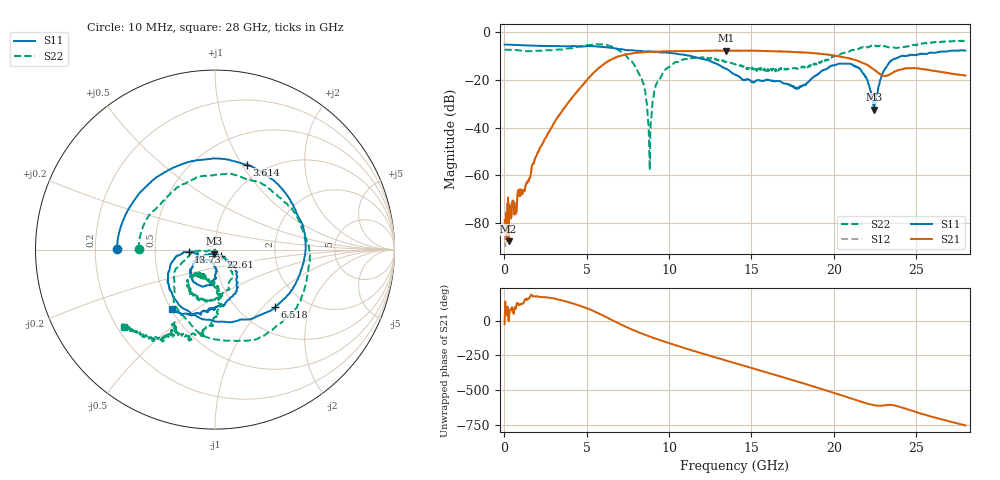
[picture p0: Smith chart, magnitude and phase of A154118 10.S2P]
!  2-Port S-parameters saved by WinCal
! VAR MeasName=S-Parameters (CALIBRATED_DATA) read from VNA (N5230A)
! VAR MeasDate=2015-9-10 14:35:09
! VAR NAME=A154118 10
! VAR FILENAME=A154118 10.S2P
! VAR DATE=2015-9-10 14:35:09
! VAR PHYS_PORTS=1,2
# Hz S DB R 50
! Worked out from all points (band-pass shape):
!   801 points, 10 MHz to 28 GHz, reference 50 ohm
!   highest |S21| = -7.79 dB at 13.45 GHz (marker M1); lowest = -87.6 dB at 254.9 MHz (marker M2)
!   |S21| within 3 dB of the highest: 6.716 GHz to 20.77 GHz (14.05 GHz wide, 102 % of centre)
!   lowest |S11| = -32.6 dB at 22.44 GHz (marker M3), VSWR 1.05, Z = 49.3 - j2.21 ohm
!   |S11| at or under -10 dB: 11.27 GHz to 24.14 GHz (12.87 GHz wide, 72.7 % of centre); 24.27452 GHz to 24.36083 GHz (86.3 MHz wide, 0.355 % of centre); 24.36195 GHz to 24.42704 GHz (65.09 MHz wide, 0.267 % of centre)
!   |S22| runs from -57.8 to -3.5 dB; largest |S21 - S12| = 0.0071
!   S11 on the Smith chart (normalised r, x): 10 MHz: 0.30, +0.00; 3.614 GHz: 0.83, +1.05; 6.518 GHz: 1.44, -1.17; 13.73 GHz: 0.74, -0.02; 22.61 GHz: 1.06, -0.08; 28 GHz: 0.51, -0.40
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1e7  -5.29 179.6  -78.78 -25.4  -79.54 -24.8  -7.49 179.8
2.549125e8  -5.29 172.2  -87.62 -2.1  -75.94 71.4  -7.44 172.1
3.613712e9  -5.94 69.5  -32.06 143.0  -32.03 143.0  -7.25 62.7
4.698325e9  -6.04 27.7  -22.61 103.5  -22.56 103.3  -6.00 12.5
5.573012e9  -6.03 -7.9  -16.06 60.8  -16.04 60.8  -5.06 -35.4
6.517675e9  -6.68 -43.8  -11.44 5.3  -11.43 5.1  -6.08 -91.9
8.302038e9  -7.94 -90.1  -8.59 -90.9  -8.52 -91.1  -19.42 -176.6
8.82685e9  -8.12 -100.8  -8.36 -114.7  -8.28 -114.9  -57.83 -47.6
9.10675e9  -8.32 -106.8  -8.26 -126.8  -8.21 -127.2  -24.36 -42.6
9.351662e9  -8.46 -111.7  -8.27 -136.9  -8.20 -137.2  -20.75 -39.0
1.089111e10  -9.52 -139.5  -8.02 163.5  -7.98 162.7  -11.50 -83.1
1.34452e10  -15.29 -175.3  -7.79 72.9  -7.77 72.4  -12.63 -130.1
1.37251e10  -16.60 -174.8  -7.82 63.1  -7.82 62.3  -12.86 -131.5
1.4005e10  -17.83 -175.1  -7.84 53.4  -7.81 53.0  -13.50 -132.7
1.603428e10  -20.12 -142.0  -8.03 -17.7  -7.98 -18.4  -16.43 -115.7
1.869332e10  -19.18 -87.1  -8.81 -112.2  -8.86 -112.5  -13.38 -88.2
2.110746e10  -13.66 -128.0  -11.36 157.0  -11.38 155.7  -7.49 -91.7
2.191218e10  -18.77 -153.6  -13.36 126.4  -13.42 125.9  -6.27 -97.1
2.243699e10  -32.58 -107.2  -15.69 109.9  -15.77 109.8  -5.73 -104.6
2.261192e10  -26.02 -49.9  -16.58 106.6  -16.57 106.3  -5.79 -108.8
2.334666e10  -13.00 -55.4  -17.97 112.0  -17.94 111.9  -6.42 -118.0
2.8e10  -7.82 -126.1  -18.23 -36.7  -18.25 -37.4  -3.55 -139.5
